PROGRAM MAIN_CM

VAR CONSTANT
	cInitDFT 			: ST_CM_SparseSpectrum_InitPars := ( 	nWindowLength 		:= cWindowLength,
																fSampleRate			:= cSampleRate,
																nBins				:= cDFTBins,
																eSpectrumType		:= E_CM_SpectrumType.eCM_DFT,
																eWindowType 		:= E_CM_WindowType.eCM_RectangularWindow, 
																eScalingType 		:= E_CM_ScalingType.eCM_NoScaling,
																bTransformToDecibel	:= FALSE );

	cInitMagnitude		: ST_CM_SparseSpectrum_InitPars := ( 	nWindowLength 		:= cWindowLength,
																fSampleRate			:= cSampleRate,
																nBins				:= cDFTBins,
																eSpectrumType		:= E_CM_SpectrumType.eCM_Magnitude,
																eWindowType 		:= E_CM_WindowType.eCM_HannWindow, 
																eScalingType 		:= E_CM_ScalingType.eCM_PeakAmplitude,
																bTransformToDecibel	:= FALSE );
														
	cInitPower 			: ST_CM_SparseSpectrum_InitPars := ( 	nWindowLength 		:= cWindowLength,
																fSampleRate			:= cSampleRate,
																nBins				:= cDFTBins,
																eSpectrumType		:= E_CM_SpectrumType.eCM_Power,
																eWindowType 		:= E_CM_WindowType.eCM_HannWindow, 
																eScalingType 		:= E_CM_ScalingType.eCM_PeakAmplitude,
																bTransformToDecibel	:= FALSE );

	cInitRealFFT		: ST_CM_RealFFT_InitPars := ( nFFT_Length := cWindowLength, bForward := TRUE, bHalfSpec := TRUE);

	cInitMagSpec		: ST_CM_MagnitudeSpectrum_InitPars := ( nFFT_Length			:= cWindowLength,
																nWindowLength		:= cWindowLength,
																eWindowType 		:= E_CM_WindowType.eCM_HannWindow, 
																eScalingType 		:= E_CM_ScalingType.eCM_PeakAmplitude,
																bTransformToDecibel	:= FALSE );
	
	cInitPowerSpec		: ST_CM_PowerSpectrum_InitPars := ( 	nFFT_Length			:= cWindowLength,
																nWindowLength		:= cWindowLength,
																eWindowType 		:= E_CM_WindowType.eCM_HannWindow, 
																eScalingType 		:= E_CM_ScalingType.eCM_PeakAmplitude,
																bTransformToDecibel	:= FALSE );
END_VAR

VAR
	// Sparse algorithms
	fbDFT			: FB_CMA_SparseSpectrum :=(	stInitPars := cInitDFT, nOwnID := eID_SparseSpectrum_DFT, aDestIDs := [eID_Sink_DFT] );
	fbMagnitude		: FB_CMA_SparseSpectrum :=(	stInitPars := cInitMagnitude, nOwnID := eID_SparseSpectrum_Magnitude, aDestIDs := [eID_Sink_Magnitude] );
	fbPower			: FB_CMA_SparseSpectrum :=(	stInitPars := cInitPower, nOwnID := eID_SparseSpectrum_Power, aDestIDs := [eID_Sink_Power] );
	
	// Reference algorithms
	fbRealFFT			: FB_CMA_RealFFT 			:= ( stInitPars := cInitRealFFT, nOwnID := eID_RealFFT, aDestIDs := [eID_Sink_RealFFT] );
	fbMagnitudeSpectrum	: FB_CMA_MagnitudeSpectrum	:= ( stInitPars := cInitMagSpec, nOwnID := eID_MagnitudeSpectrum, aDestIDs := [eID_Sink_MagnitudeSpectrum] );
	fbPowerSpectrum		: FB_CMA_PowerSpectrum		:= ( stInitPars := cInitPowerSpec, nOwnID := eID_PowerSpectrum, aDestIDs := [eID_Sink_PowerSpectrum] );
	
	// Configuration
	bConfigure		: BOOL := TRUE;			
	aDFTBins		: ARRAY [1..cDFTBins] OF UDINT;
	i				: UDINT;
	k				: DINT;
	nyquist			: DINT := UDINT_TO_DINT(cWindowLength/2);
	
	fbErrHist		: FB_HRErrHist; // error monitoring
END_VAR

// Configuration
IF bConfigure THEN
	// Compute parameters, adjust if cDFTBins is changed.
	FOR i := 1 TO cBands DO
		k := LREAL_TO_DINT(cSetFrequency[i] / cResolution);
		aDFTBins[(i-1) * cBandWidth + 1] := DINT_TO_UDINT(MAX(k - 2, 1));
		aDFTBins[(i-1) * cBandWidth + 2] := DINT_TO_UDINT(MAX(k - 1, 1));
		aDFTBins[(i-1) * cBandWidth + 3] := DINT_TO_UDINT(MIN(k + 0, nyquist));
		aDFTBins[(i-1) * cBandWidth + 4] := DINT_TO_UDINT(MIN(k + 1, nyquist));
		aDFTBins[(i-1) * cBandWidth + 5] := DINT_TO_UDINT(MIN(k + 2, nyquist));
	END_FOR
	
	// Configure DFT
	fbDFT.Configure(pArg := ADR(aDFTBins), nArgSize := SIZEOF(aDFTBins));
	IF fbDFT.bError THEN
		fbErrHist.AddError(bErr:=TRUE, hrErrCode:=fbDFT.hrErrorCode, sErrSource:='MAIN_CM.fbDFT.Configure'); // error monitoring
		// ToDo: if error
	END_IF
	
	// Configure Magnitude
	fbMagnitude.Configure(pArg := ADR(aDFTBins), nArgSize := SIZEOF(aDFTBins));
	IF fbMagnitude.bError THEN
		fbErrHist.AddError(bErr:=TRUE, hrErrCode:=fbMagnitude.hrErrorCode, sErrSource:='MAIN_CM.fbMagnitude.Configure'); // error monitoring
		// ToDo: if error
	END_IF
	
	// Configure Power
	fbPower.Configure(pArg := ADR(aDFTBins), nArgSize := SIZEOF(aDFTBins));
	IF fbPower.bError THEN
		fbErrHist.AddError(bErr:=TRUE, hrErrCode:=fbPower.hrErrorCode, sErrSource:='MAIN_CM.fbPower.Configure'); // error monitoring
		// ToDo: if error
	END_IF
	
	bConfigure := FALSE;
END_IF

// Call DFT
fbDFT.Call();
IF fbDFT.bError THEN
	fbErrHist.AddError(bErr:=TRUE, hrErrCode:=fbDFT.hrErrorCode, sErrSource:='MAIN_CM.fbDFT'); // error monitoring
	// ToDo: if error
END_IF

// Call Magnitude
fbMagnitude.Call();
IF fbMagnitude.bError THEN
	fbErrHist.AddError(bErr:=TRUE, hrErrCode:=fbMagnitude.hrErrorCode, sErrSource:='MAIN_CM.fbMagnitude'); // error monitoring
	// ToDo: if error
END_IF

// Call Power
fbPower.Call();
IF fbPower.bError THEN
	fbErrHist.AddError(bErr:=TRUE, hrErrCode:=fbPower.hrErrorCode, sErrSource:='MAIN_CM.fbPower'); // error monitoring
	// ToDo: if error
END_IF

// Call RealFFT
fbRealFFT.Call();
IF fbRealFFT.bError THEN
	fbErrHist.AddError(bErr:=TRUE, hrErrCode:=fbRealFFT.hrErrorCode, sErrSource:='MAIN_CM.fbRealFFT'); // error monitoring
	// ToDo: if error
END_IF

// Call MagnitudeSpectrum
fbMagnitudeSpectrum.Call();
IF fbMagnitudeSpectrum.bError THEN
	fbErrHist.AddError(bErr:=TRUE, hrErrCode:=fbMagnitudeSpectrum.hrErrorCode, sErrSource:='MAIN_CM.fbMagnitudeSpectrum'); // error monitoring
	// ToDo: if error
END_IF

// Call PowerSpectrum
fbPowerSpectrum.Call();
IF fbPowerSpectrum.bError THEN
	fbErrHist.AddError(bErr:=TRUE, hrErrCode:=fbPowerSpectrum.hrErrorCode, sErrSource:='MAIN_CM.fbPowerSpectrum'); // error monitoring
	// ToDo: if error
END_IF

END_PROGRAM
